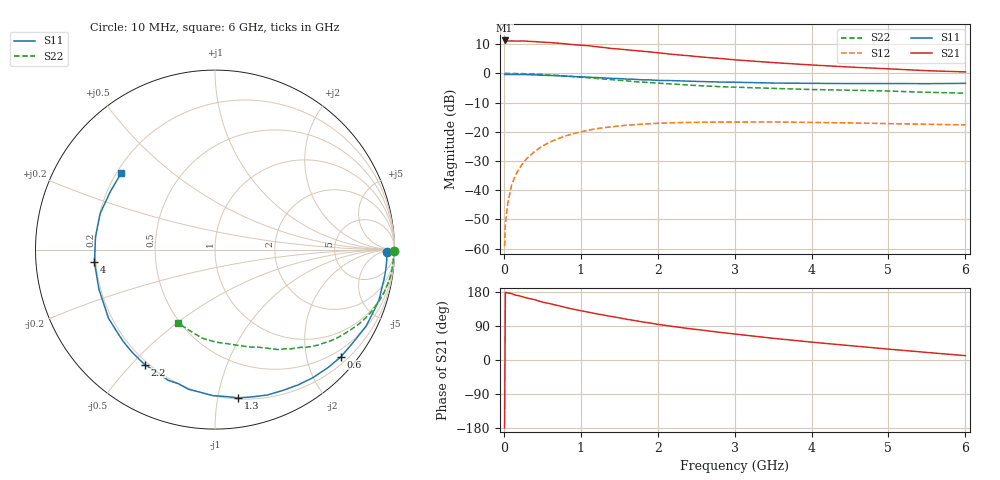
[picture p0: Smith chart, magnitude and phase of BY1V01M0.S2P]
! SIEMENS Small Signal Semiconductors
! BFY420
! Si NPN RF SIEGET Grounded Emitter Transistor in MICRO-X
! VCE = 1 V  IC = 1 mA
! Common Emitter S-Parameters:  October  1996
# GHz  S  MA  R  50
!  f  S11  S21  S12  S22
! GHz  MAG  ANG  MAG  ANG  MAG  ANG  MAG  ANG
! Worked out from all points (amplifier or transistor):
!   36 points, 10 MHz to 6 GHz, reference 50 ohm
!   highest |S21| = 11.3 dB at 10 MHz (marker M1)
!   |S21| within 3 dB of that: start of sweep to 1.52 GHz
!   unconditionally stable (mu >= 1): 4.532 GHz to end of sweep
!   at 250 MHz: K = 0.04, MSG = 20.9 dB, |S12| = -30.7 dB
!   at 1.4 GHz: K = 0.23, MSG = 13.4 dB, |S12| = -18.3 dB
!   at 6 GHz: K = 1.33, MAG = 5.6 dB, |S12| = -17.6 dB
!   S11 on the Smith chart (normalised r, x): 10 MHz: 44, -15; 600 MHz: 0.34, -2.69; 1.3 GHz: 0.21, -1.15; 2.2 GHz: 0.19, -0.55; 4 GHz: 0.19, -0.05; 6 GHz: 0.22, +0.34
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0.01  0.9598 -0.8  3.661 -179.3  0.0011 93.2  0.9987 -0.3
0.02  0.9567 -1.3  3.635 178.8  0.0026 79.2  0.9993 -0.7
0.05  0.9589 -3.5  3.583 176.9  0.0059 88.1  0.9959 -1.9
0.1  0.958 -6.9  3.6 175.1  0.0121 86.4  0.9949 -3.7
0.15  0.956 -10.2  3.572 171.3  0.0179 83.3  0.9933 -5.5
0.25  0.9561 -17.1  3.59 166.4  0.0292 78.7  0.9872 -9.2
0.4  0.9438 -26.8  3.496 159.1  0.046 73.1  0.9706 -14.5
0.5  0.9278 -33.7  3.425 152.9  0.0567 68.9  0.9562 -17.9
0.6  0.9214 -40.3  3.373 148.6  0.0668 65.2  0.9398 -21.3
0.8  0.8979 -52.7  3.201 138.9  0.0847 56.9  0.9008 -27.6
1.1  0.861 -70.2  2.977 126.1  0.1067 46.5  0.8396 -35.9
1.3  0.8363 -81.0  2.775 118.5  0.1176 40.5  0.7984 -40.7
1.6  0.7985 -96.1  2.529 107.3  0.1295 32.4  0.7427 -47.2
1.8  0.7748 -105.2  2.392 100.5  0.1349 27.8  0.7088 -50.7
2.2  0.751 -121.5  2.111 88.5  0.1429 19.4  0.6581 -57.8
2.4  0.7359 -128.5  2.007 83.0  0.1443 16.2  0.6301 -61.0
2.8  0.7105 -141.6  1.805 73.2  0.1466 10.3  0.5926 -66.5
3.5  0.6834 -161.3  1.53 57.3  0.1471 2.4  0.5529 -75.5
4  0.6752 -174.1  1.393 47.2  0.1446 -2.1  0.529 -82.4
4.5  0.6697 173.9  1.283 37.9  0.1417 -5.9  0.5153 -89.6
5.5  0.6668 151.0  1.112 20.0  0.1344 -10.0  0.4744 -106.7
6  0.6752 140.5  1.059 11.5  0.1313 -10.2  0.4576 -116.4
